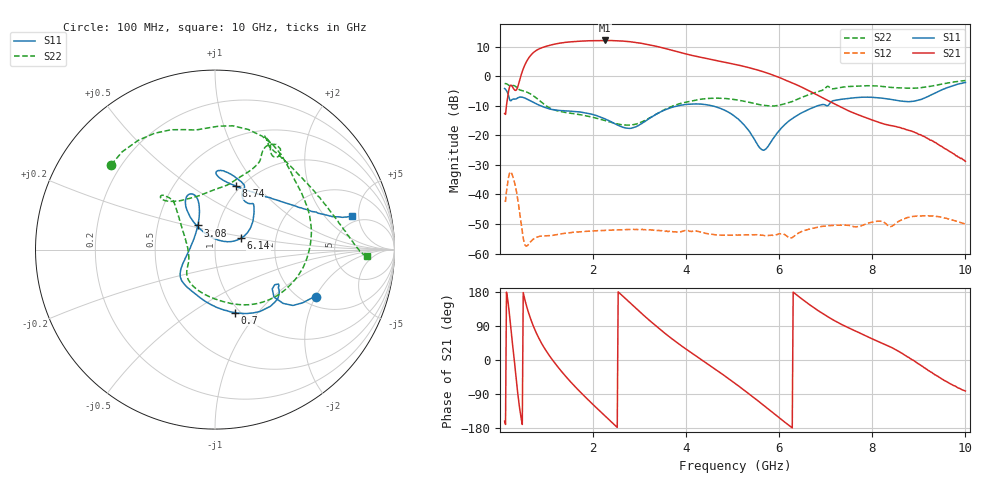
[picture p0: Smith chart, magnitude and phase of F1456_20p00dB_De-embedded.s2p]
! Integrated Device Technology
! Corporate Headquarters
! 6024 Silver Creek Valley Road
! San Jose, CA 95138  USA
! Phone:  1-408-284-8200
! Toll Free:  1-800-223-1366
! Webpage:  http://www.idt.com/
! Timing and RF Division
! 515 Groton Road, Suite 102
! Westford, MA 01886-6024
! Device:  F1456
! Description: 6-bit 0.5 dB Transmit Variable Gain Amplifier
! Frequency:  2100.0 -  2950.00 MHz
! Package:  6x6 mm Thin QFN Plastic Package: 28 pin
! State:  40
! Atten State:  20.0 dB
! Voltage:  +5.00 Volts
! Current:  216.979 mA
! Data:  The device was measured on a the F1455 evaluation board which has
!  individual transmission lines to the RF pins.  Data was collected
!  using a calibrated network analyzer.  The evaluation board was
!  de-embedded using a TRL calibration technique.
!  The reference plane is the edge of the package pin.
!  Pin  1 = CSb
!  Pin  2 = DATA
!  Pin  3 = CLK
!  Pin  4 = RSET
!  Pin  5 = GND
!  Pin  6 = RFIN  = Port 1
!  Pin  7 = GND
!  Pin  8 = NC
!  Pin  9 = NC
!  Pin 10 = NC
!  Pin 11 = NC
!  Pin 12 = NC
!  Pin 13 = NC
!  Pin 14 = /STBY
!  Pin 15 = GND
!  Pin 16 = RFOUT  = Port 2
!  Pin 17 = GND
!  Pin 18 = NC
!  Pin 19 = NC
!  Pin 20 = NC
!  Pin 21 = GND
!  Pin 22 = NC
!  Pin 23 = GND
!  Pin 24 = NC
!  Pin 25 = NC
!  Pin 26 = NC
!  Pin 27 = GND
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# GHz S dB R 50
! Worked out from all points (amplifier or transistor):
!   496 points, 100 MHz to 10 GHz, reference 50 ohm
!   highest |S21| = 12.1 dB at 2.26 GHz (marker M1)
!   |S21| within 3 dB of that: 822 MHz to 3.619 GHz (2.797 GHz wide, 126 % of centre)
!   unconditionally stable (mu >= 1): start of sweep to end of sweep
!   at 1.74 GHz: K = 48.54, MAG = 12.4 dB, |S12| = -52.6 dB
!   at 5.06 GHz: K = 123.81, MAG = 4.9 dB, |S12| = -53.8 dB
!   at 10 GHz: K = 478.85, MAG = -19.2 dB, |S12| = -50.0 dB
!   S11 on the Smith chart (normalised r, x): 100 MHz: 2.36, -2.00; 700 MHz: 0.94, -0.76; 3.08 GHz: 0.80, +0.22; 6.14 GHz: 1.32, +0.17; 8.74 GHz: 0.95, +0.78; 10 GHz: 4.17, +4.09
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0.1  -4.16 -25.0  -12.64 -161.6  -42.29 49.2  -2.53 140.8
0.22  -8.25 -34.5  -3.11 100.8  -32.35 -51.0  -3.42 99.1
0.3  -7.72 -30.6  -4.39 9.2  -35.20 -134.6  -3.17 74.7
0.42  -7.08 -37.5  -1.56 -125.2  -45.81 140.8  -4.59 41.3
0.56  -7.57 -56.5  4.64 147.4  -57.49 148.3  -5.23 10.8
0.7  -8.70 -72.7  7.73 94.9  -55.34 143.0  -6.42 -20.4
0.94  -10.41 -96.8  9.86 34.4  -54.04 99.3  -9.42 -65.1
1.16  -11.37 -114.1  10.80 -5.0  -53.74 74.9  -11.34 -92.4
1.48  -11.78 -131.5  11.58 -52.5  -52.97 50.3  -12.44 -119.3
1.76  -12.19 -142.0  11.89 -88.8  -52.59 33.4  -13.12 -133.5
2.26  -14.46 -158.2  12.10 -148.0  -52.13 9.1  -15.01 -149.0
2.64  -17.27 174.1  11.89 168.3  -51.94 -8.1  -16.45 -165.8
3.08  -15.63 125.6  11.02 118.8  -51.91 -28.7  -15.19 161.3
3.4  -12.48 111.5  9.97 84.9  -52.16 -43.6  -12.46 142.9
4.1  -9.40 113.6  7.13 20.2  -52.47 -74.4  -8.43 131.2
5.06  -13.74 127.8  3.98 -62.5  -53.75 -121.7  -7.94 136.2
5.66  -25.05 71.2  1.50 -119.1  -53.84 -159.4  -9.83 119.4
6.14  -16.08 23.4  -1.36 -166.0  -53.83 167.5  -9.22 85.3
6.7  -10.78 41.7  -5.40 141.8  -51.51 145.2  -5.90 64.6
8.36  -7.75 88.0  -16.59 36.5  -50.84 70.0  -3.73 62.5
8.74  -8.55 72.0  -18.13 9.7  -47.92 66.6  -4.05 49.2
10  -2.10 13.9  -28.81 -81.8  -50.02 -22.5  -1.46 -2.6
